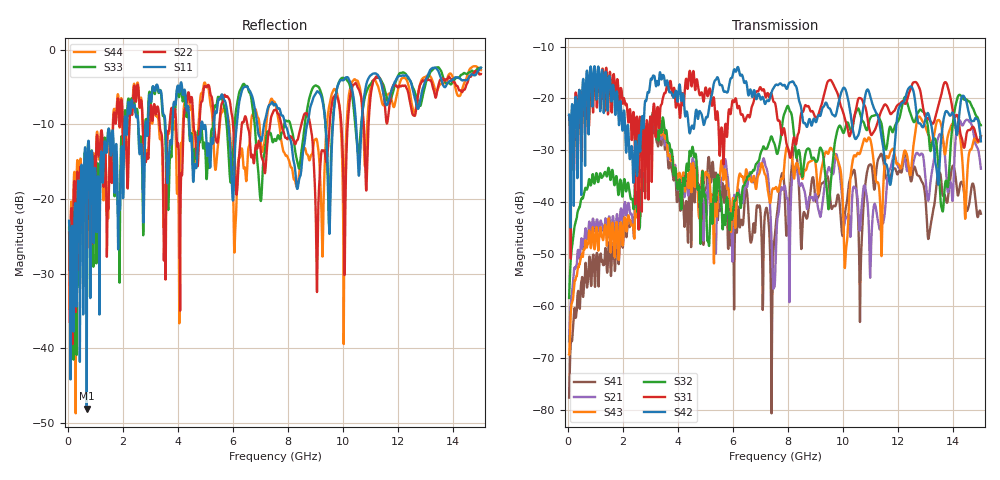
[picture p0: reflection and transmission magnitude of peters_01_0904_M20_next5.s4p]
# MHZ S RI R 50.00
! FREQ  S11  S12  S13  S14
!  S21  S22  S23  S24
!  S31  S32  S33  S34
!  S41  S42  S43  S44
!  REAL  IMAG  REAL  IMAG  REAL  IMAG  REAL  IMAG
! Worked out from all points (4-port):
!   1496 points, 50 MHz to 15 GHz, reference 50 ohm
!   strongest paths, dB at 50 MHz, 3.79 GHz, 7.53 GHz, 11.27 GHz, 15 GHz:
!     S42: -23.1, -19.2, -17.5, -23.6, -28.3
!     S31: -23.3, -19.4, -20.9, -24.3, -27.3
!     S32: -58.5, -30.5, -29.2, -23.3, -25.2
!     S43: -69.3, -31.2, -37.3, -36.3, -27.3
!     S21: -66.8, -32.0, -54.4, -43.8, -33.5
!     S41: -77.7, -33.9, -45.9, -31.7, -42.2
!   lowest |S11| = -48.1 dB at 690 MHz (marker M1), VSWR 1.01, Z = 49.9 - j0.383 ohm
!   |S11| at or under -10 dB: start of sweep to 2.062 GHz; 4.415 GHz to 4.848 GHz (432.8 MHz wide, 9.34 % of centre); 7.891 GHz to 8.692 GHz (800.7 MHz wide, 9.66 % of centre)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
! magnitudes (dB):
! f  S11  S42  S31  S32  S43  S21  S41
! 50 MHz  -22.9  -23.1  -23.3  -58.5  -69.3  -66.8  -77.7
! 690 MHz  -48.1  -14.7  -17.4  -37.6  -48.8  -47.0  -55.5
! 3.12 GHz  -5.0  -15.6  -21.1  -22.9  -23.0  -24.9  -25.9
! 5.11 GHz  -12.5  -22.6  -18.9  -47.6  -34.8  -35.6  -31.4
! 7.14 GHz  -9.8  -20.8  -18.6  -29.6  -34.4  -32.0  -43.6
! 7.49 GHz  -7.5  -17.8  -20.7  -28.5  -37.4  -56.3  -47.7
! 15 GHz  -2.4  -28.3  -27.3  -25.2  -27.3  -33.5  -42.2
